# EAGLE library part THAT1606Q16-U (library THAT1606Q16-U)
THAT CORPORATION - THAT1606Q16-U - LINE DRIVER, BALANCED, SMD, 1606 Source: Datasheet
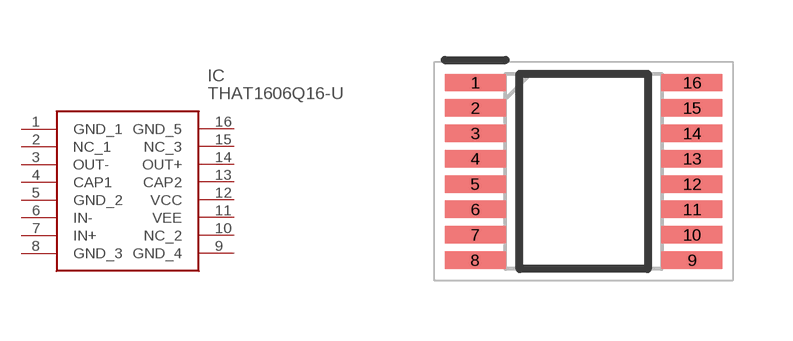
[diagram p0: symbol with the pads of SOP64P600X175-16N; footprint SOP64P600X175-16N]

Designator prefix IC

## THAT1606Q16-U (Description: THAT CORPORATION - THAT1606Q16-U - LINE DRIVER, BALANCED, SMD, 1606; Height: 1.75mm; Manufacturer_Name: THAT CORPORATION; Manufacturer_Part_Number: THAT1606Q16-U)  [SOP64P600X175-16N]
1  GND_1
2  NC_1
3  OUT-
4  CAP1
5  GND_2
6  IN-
7  IN+
8  GND_3
9  GND_4
10  NC_2
11  VEE
12  VCC
13  CAP2
14  OUT+
15  NC_3
16  GND_5

## Footprint SOP64P600X175-16N (pad centres in mm)
16 pin QSOP
smd 1.525 x 0.435: 1 -2.712,2.222; 2 -2.712,1.588; 3 -2.712,0.952; 4 -2.712,0.318; 5 -2.712,-0.318; 6 -2.712,-0.952; 7 -2.712,-1.588; 8 -2.712,-2.222; 9 2.712,-2.222; 10 2.712,-1.588; 11 2.712,-0.952; 12 2.712,-0.318; 13 2.712,0.318; 14 2.712,0.952; 15 2.712,1.588; 16 2.712,2.222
